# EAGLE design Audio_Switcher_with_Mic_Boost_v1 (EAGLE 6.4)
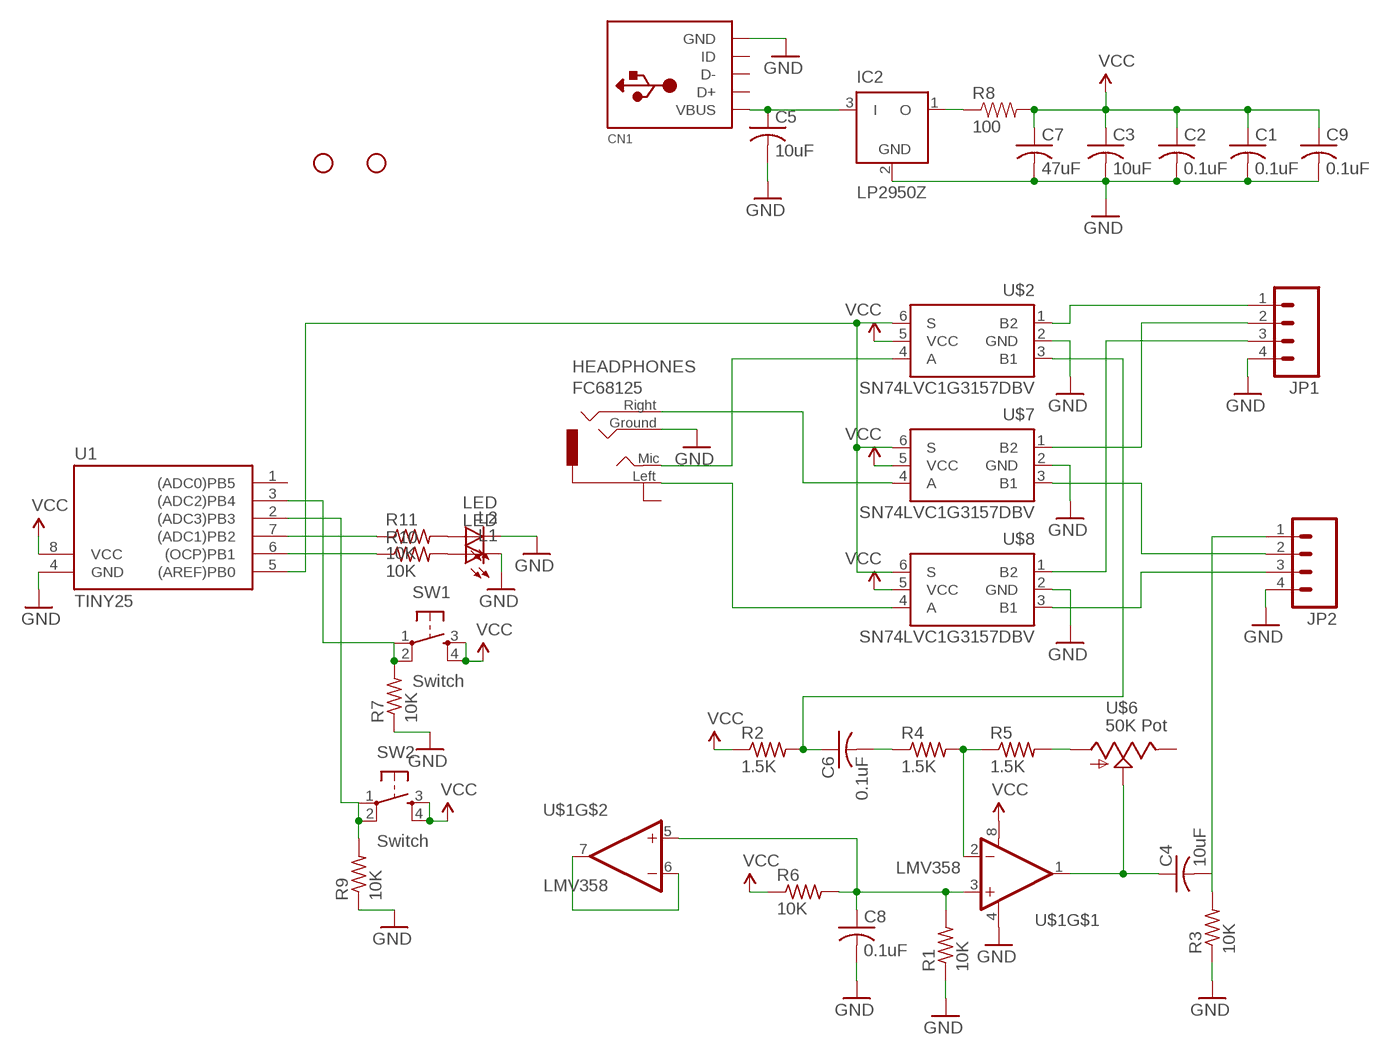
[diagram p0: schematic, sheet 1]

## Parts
C1  0.1uF  C-USC0805K  [C0805K]
C2  0.1uF  C-USC0805K  [C0805K]
C3  10uF  C-US025-024X044  [C025-024X044]
C4  10uF  C-US025-024X044  [C025-024X044]
C5  10uF  C-US025-024X044  [C025-024X044]
C6  0.1uF  C-USC0805K  [C0805K]
C7  47uF  C-US025-024X044  [C025-024X044]
C8  0.1uF  C-USC0805K  [C0805K]
C9  0.1uF  C-USC0805K  [C0805K]
CN1  USBMINIB  [USB-MINIB]
HEADPHONES  FC68125  [FC68125]
IC2  LP2950Z  [TO92]
JP1  M04PTH  [1X04]
JP2  M04PTH  [1X04]
JP3  STAND-OFF2MM  [STAND-OFF-M2]
JP5  STAND-OFF2MM  [STAND-OFF-M2]
L1  LED  LED3MM  [LED3MM]
L2  LED  LED3MM  [LED3MM]
R1  10K  R-US_R0805_2  [R0805_2]
R2  1.5K  R-US_R0805_2  [R0805_2]
R3  10K  R-US_R0805_2  [R0805_2]
R4  1.5K  R-US_R0805_2  [R0805_2]
R5  1.5K  R-US_R0805_2  [R0805_2]
R6  10K  R-US_R0805_2  [R0805_2]
R7  10K  R-US_R0805_2  [R0805_2]
R8  100  RESISTOR5MM  [RESISTOR5MM]
R9  10K  R-US_R0805_2  [R0805_2]
R10  10K  R-US_R0805_2  [R0805_2]
R11  10K  R-US_R0805_2  [R0805_2]
SW1  Switch  TAC_SWITCHPTH  [TACTILE-PTH]
SW2  Switch  TAC_SWITCHPTH  [TACTILE-PTH]
U1  TINY25  [SO08]
U$1  LMV358  LM358SO-08  [SO-08]
U$2  SN74LVC1G3157DBV  [SOT23-DBV-2]
U$6  50K Pot  POT  [ENC_9.6MM]
U$7  SN74LVC1G3157DBV  [SOT23-DBV-2]
U$8  SN74LVC1G3157DBV  [SOT23-DBV-2]

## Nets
GND: C1.2 C2.2 C3.2 C5.2 C7.2 C8.2 C9.2 CN1.GND HEADPHONES.4 IC2.2(GND) JP1.4 JP2.4 L1.K(C) L2.K(C) R1.1 R3.1 R7.1 R9.1 U1.4(GND) U$1.4(V-) U$2.2(GND) U$7.2(GND) U$8.2(GND)
INPUT_LEFT: HEADPHONES.1 U$8.4(A)
INPUT_MIC: HEADPHONES.3 U$2.4(A)
INPUT_RIGHT: HEADPHONES.2 U$7.4(A)
N$1: C4.1 U$1.1(OUT) U$6.C(S)
N$2: C6.1 R2.2 U$2.3(B1)
N$3: JP1.2 U$7.1(B2)
N$4: JP2.2 U$7.3(B1)
N$5: JP2.3 U$8.3(B1)
N$6: JP1.3 U$8.1(B2)
N$7: R5.2 U$6.A
N$10: JP1.1 U$2.1(B2)
N$11: R10.1 U1.6((OCP)PB1)
N$13: R11.1 U1.7((ADC1)PB2)
N$14: L1.A R10.2
N$15: L2.A R11.2
N$16: C8.1 R1.2 R6.2 U$1.3(+IN) U$1.5(+IN)
N$18: R4.2 R5.1 U$1.2(-IN)
N$19: C6.2 R4.1
N$21: C4.2 JP2.1 R3.2
N$22: C5.1 CN1.VBUS IC2.3(I)
N$23: U$1.6(-IN) U$1.7(OUT)
N$24: IC2.1(O) R8.P$1
SELECT: U1.5((AREF)PB0) U$2.6(S) U$7.6(S) U$8.6(S)
SW2: R9.2 SW2.1 SW2.2 U1.2((ADC3)PB3)
VCC: C1.1 C2.1 C3.1 C7.1 C9.1 R2.1 R6.1 R8.P$2 SW1.3 SW1.4 SW2.3 SW2.4 U1.8(VCC) U$1.8(V+) U$2.5(VCC) U$7.5(VCC) U$8.5(VCC)
VCC1: R7.2 SW1.1 SW1.2 U1.3((ADC2)PB4)
Unconnected: CN1.D+ CN1.D- CN1.ID HEADPHONES.5 U1.1((ADC0)PB5) U$6.B(E)

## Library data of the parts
C1-C9 = adafruit:C-US: CAPACITOR, American symbol
CN1 = adafruit:USB: USB Connectors USBMINIB - Surface Mount Female Mini-B USB Connector 4UConnector: 06564 By microbuilder.eu Thru-hole RA Female Mini-B USB Connector 4UConnector: 18732 By ladyada.net
HEADPHONES = SparkFun:FC68125
IC2 = linear:LP2950: 100 mA, Low Power Low Dropout Voltage Regulator Source: http://www.onsemi.com/pub/Collateral/LP2950-D.PDF
JP1 JP2 = SparkFun:M04: Header 4 Standard 4-pin 0.1" header. Use with straight break away headers (SKU : PRT-00116), right angle break away headers (PRT-00553), swiss pins (PRT-00743), machine pins (PRT-00117), and female headers (PRT-00115). Molex polarized connector foot print use with SKU : PRT-08231 with associated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
JP3 JP5 = SparkFun:STAND-OFF: Stand Off
L1 L2 = SparkFun:LED: LEDs
R1-R7 R9-R11 = adafruit:R-US_: RESISTOR, American symbol
R8 = SparkFun:RESISTOR: Resistor
SW1 SW2 = SparkFun:TAC_SWITCH: Momentary Switch Button commonly used for reset or general input. Spark Fun Electronics SKU : COM-00097
U1 = avr-5:TINY25
U$1 = SparkFun:LM358
U$2 U$7 U$8 = texas:SN74LVC1G3157
U$6 = switch-alps_old:POT

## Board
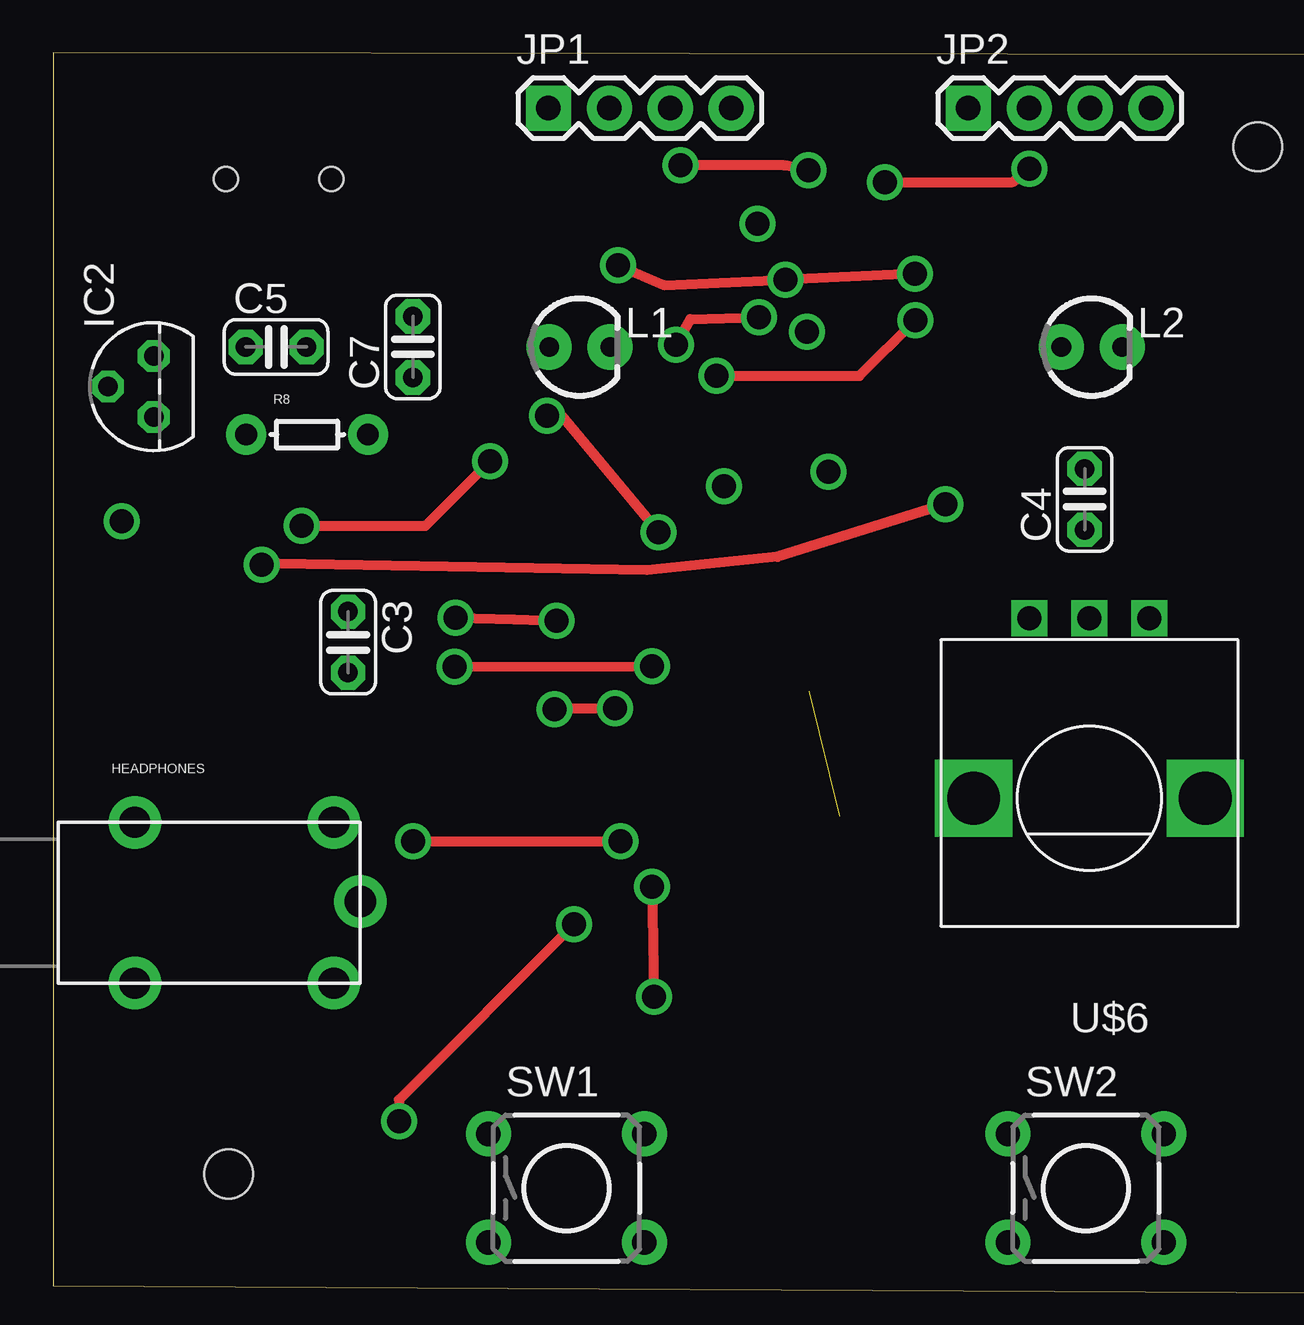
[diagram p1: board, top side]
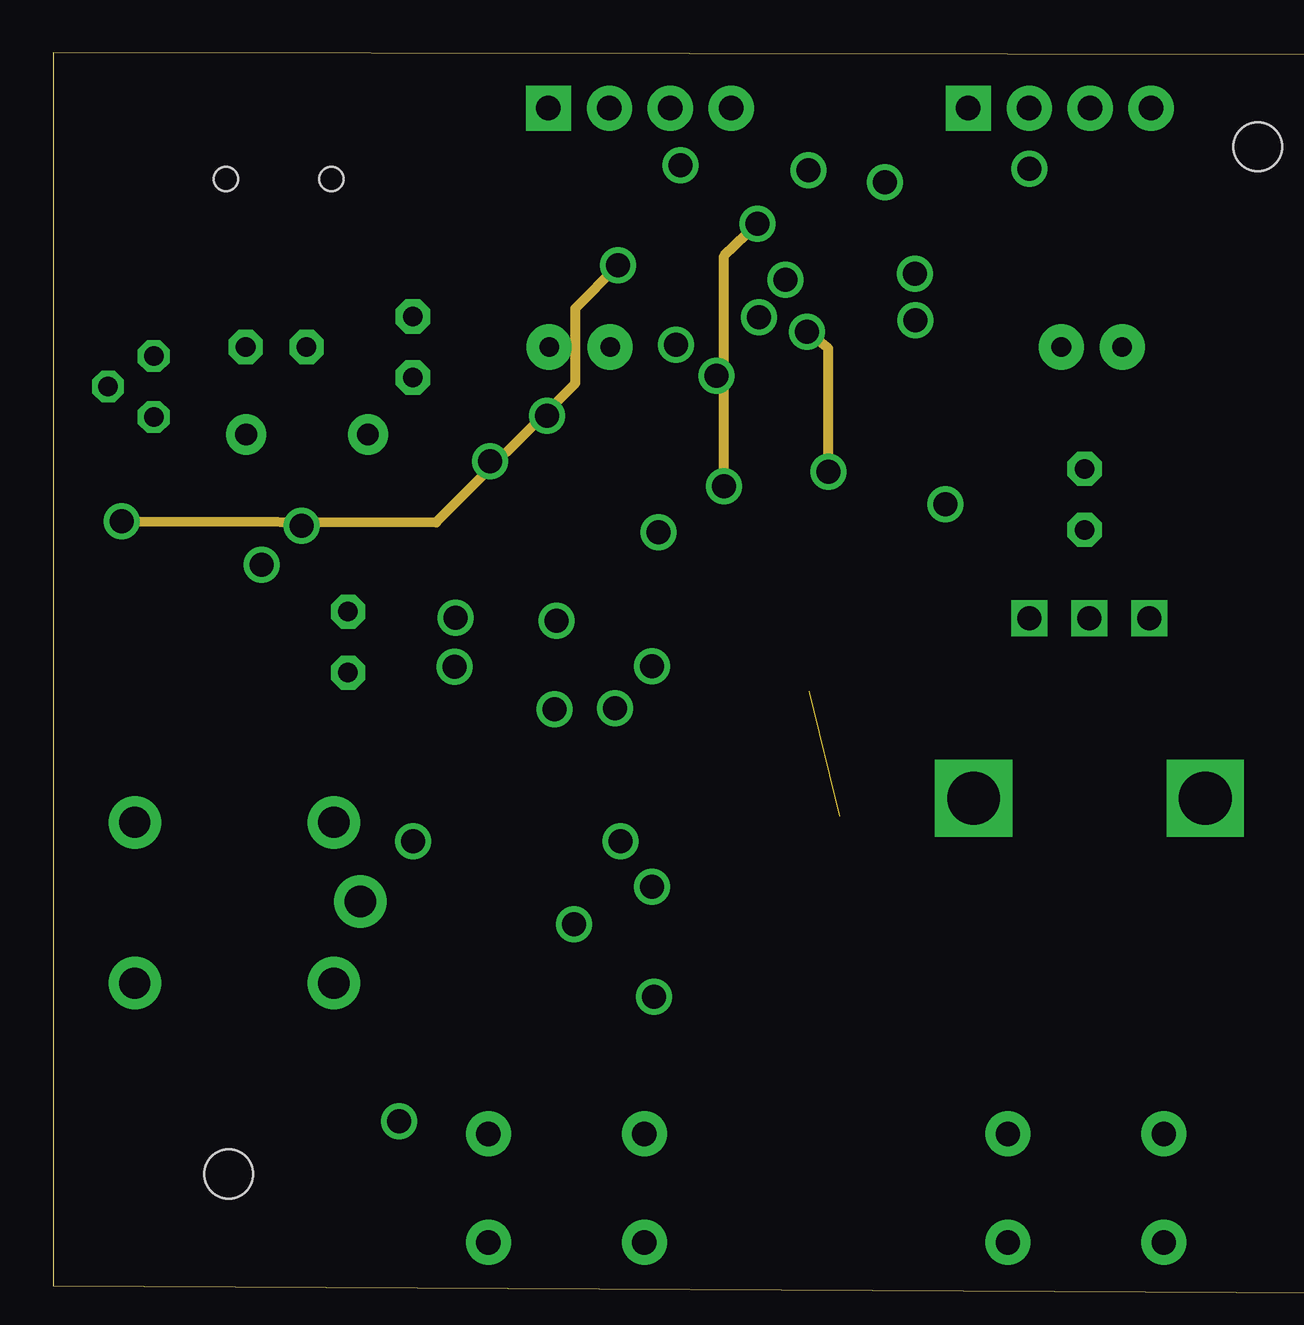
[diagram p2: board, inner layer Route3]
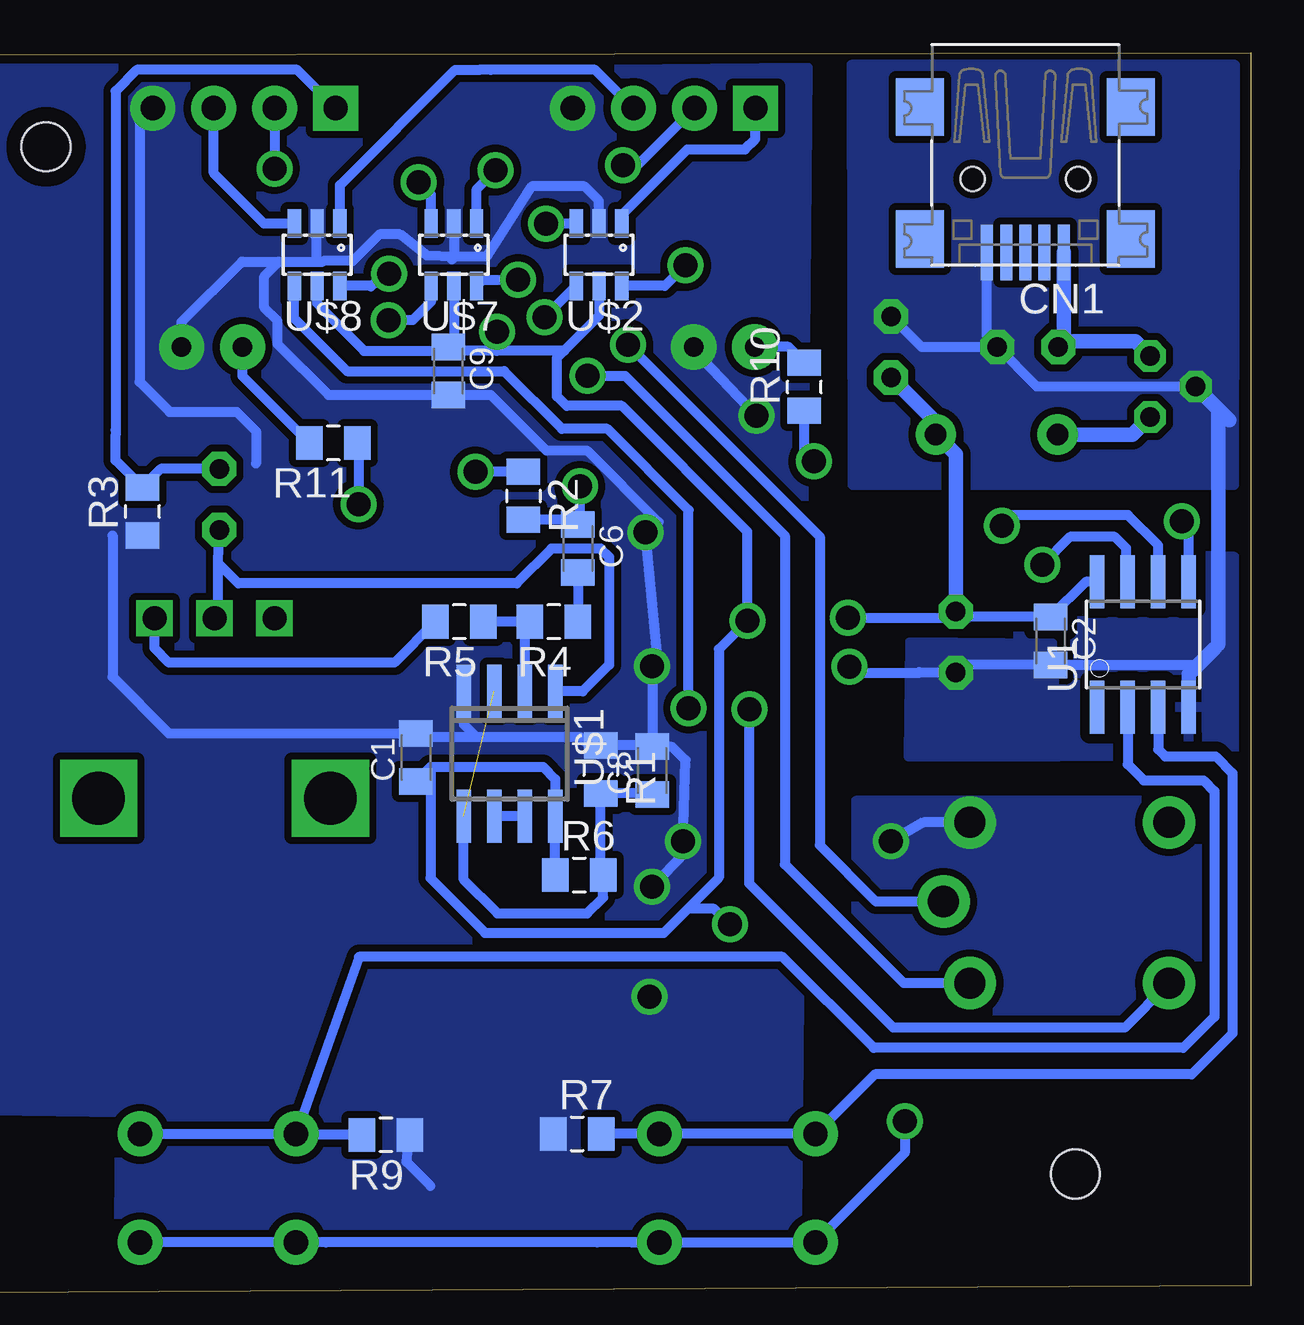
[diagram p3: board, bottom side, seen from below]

No outline drawn. Coordinates in mm, seen from the top.
Copper layers (1*16): Top 0.035mm / dielectric 1.5mm / Bottom 0.035mm
Design rules "ITead_rule": minimum track width 6mil, minimum drill 12mil, track to track 6mil, track to pad 6mil, pad to pad 6mil, via to via 6mil, smd to smd 0mil, copper to edge 10mil, drill to drill 10mil, minimum pad ring 10mil, minimum via ring 6mil, stop-mask expansion 2mil, vias tented up to drill 100mil, thermal gap 10mil
Milling: 4 lines

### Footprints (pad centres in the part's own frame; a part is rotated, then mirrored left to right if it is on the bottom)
C0805K = smd 1.1 x 1.4: 1 -1,0; 2 1,0
C025-024X044 = drill 0.813 pad 1.422 octagon: 1 -1.27,0; 2 1.27,0
USB-MINIB = smd 0.5 x 2.308: D+ 0,4.064; D- -0.8,4.064; GND 1.6,4.064; ID 0.8,4.064; VBUS -1.6,4.064 | smd 2 x 2.4: GND1 -4.4,-2; GND2 -4.4,3.5; GND3 4.4,3.5; GND4 4.4,-2 | hole 1: -2.2,1; 2.2,1
FC68125 = drill 1.3 pad 2.184: 1 -2.84,-3.66; 2 5.46,-3.66; 3 6.56,-0.26; 4 5.46,3.04; 5 -2.84,3.04
TO92 = drill 0.813 octagon: 1 -1.27,0; 2 0,1.905; 3 1.27,0
1X04 = drill 1.016 pad 1.88 square: 1 0,0 | drill 1.016 pad 1.88: 2 2.54,0; 3 5.08,0; 4 7.62,0
STAND-OFF-M2 = hole 2.032: 0,0
LED3MM = drill 0.813 pad 1.88: A -1.27,0; K 1.27,0
R0805_2 = smd 1.1 x 1.4: 1 -1,0; 2 1,0
RESISTOR5MM = drill 0.9 pad 1.676: P$1 -2.5,0; P$2 2.58,0
TACTILE-PTH = drill 1.016 pad 1.88: 1 -3.251,2.261; 2 3.251,2.261; 3 -3.251,-2.261; 4 3.251,-2.261
SO08 = smd 0.61 x 2.21: 1 -1.905,-2.616; 2 -0.635,-2.616; 3 0.635,-2.616; 4 1.905,-2.616; 5 1.905,2.616; 6 0.635,2.616; 7 -0.635,2.616; 8 -1.905,2.616
SO-08 = smd 0.6 x 2.2: 1 -1.905,-2.6; 2 -0.635,-2.6; 3 0.635,-2.6; 4 1.905,-2.6; 5 1.905,2.6; 6 0.635,2.6; 7 -0.635,2.6; 8 -1.905,2.6
SOT23-DBV-2 = smd 0.55 x 1.2: 1 -0.95,-1.3; 2 0,-1.3; 3 0.95,-1.3; 4 0.95,1.3; 5 0,1.3; 6 -0.95,1.3
ENC_9.6MM = drill 1 square: A -2.5,-7.5; B 2.5,-7.5; C 0,-7.5 | drill 2.2 square: GND1 -4.83,0; GND2 4.83,0

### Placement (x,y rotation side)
C1  34.78,-29.24 90 bottom
C2  8.33,-24.39 270 bottom
C3  12.28,-24.44 270 top
C4  42.98,-18.49 90 top
C5  9.28,-12.14 0 top
C6  28.03,-20.54 270 bottom
C7  14.98,-12.14 90 top
C8  24.93,-29.79 90 bottom
C9  33.43,-13.14 270 bottom
CN1  9.38,-4.14 180 bottom
HEADPHONES  6.23,-34.99 0 top
IC2  4.18,-13.79 90 top
JP1  20.63,-2.19 0 top
JP2  38.13,-2.19 0 top
JP3  7.3,-46.6 0 top
JP5  50.2,-3.8 0 top
L1  21.93,-12.14 0 top
L2  43.28,-12.14 0 top
R1  27.08,-29.74 270 bottom
R2  30.3,-18.34 270 bottom
R3  46.18,-18.99 90 bottom
R4  29.03,-23.59 180 bottom
R5  32.98,-23.59 180 bottom
R6  27.98,-34.14 0 bottom
R7  28.06,-44.93 0 bottom
R8  10.53,-15.79 0 top
R9  36.04,-44.97 180 bottom
R10  18.59,-13.8 90 bottom
R11  38.23,-16.14 180 bottom
SW1  21.38,-47.19 0 top
SW2  43.03,-47.19 0 top
U1  4.48,-24.54 0 bottom
U$1  30.88,-29.09 180 bottom
U$2  27.15,-8.3 180 bottom
U$6  43.18,-30.94 180 top
U$7  33.2,-8.3 180 bottom
U$8  38.9,-8.3 180 bottom

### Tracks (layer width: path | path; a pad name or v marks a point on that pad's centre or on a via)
GND  (via drill 1)
  Top 0.406: v16.71,-25.47 v24.95,-25.44 | v14.99,-32.73 v23.64,-32.73 | v20.58,-15 21.17,-15.01 v25.21,-19.86 | v24.95,-34.63 v25.04,-39.21
  Bottom 0.406: C5.2 10.98,-11.71 CN1.GND | IC2.2 8.9,-13.79 C5.2 | C7.2 13.71,-12.14 C5.2 | 47.43,-19.99 47.43,-25.89 45.08,-28.24 C1.2 | R1.1 27.58,-28.75 | U$1.4 32.78,-27.86 32.25,-28.4 | 35.18,-28.24 C1.2 | 2.58,-25.79 U1.4 | 13.78,-25.71 C3.2 11.96,-25.39 C2.2 2.18,-25.39 1.5,-24.71 | C8.2 24.98,-28.75 27.58,-28.75 | 34.18,-47.09 35.18,-46.09 R9.1 | HEADPHONES.4 13.62,-31.95 v14.99,-32.73 | 13.8,-25.69 13.78,-25.71 | L1.K 23.2,-12.25 v20.58,-15 | 33.2,-8.38 31.84,-8.38 29.96,-5.45 27.75,-5.45 27.15,-6.05 U$2.2 | 33.28,-8.5 33.2,-8.38 | 40.5,-8.58 42.03,-8.58 44.55,-11.1 L2.K | 40.5,-8.58 38.95,-8.58 | 38.95,-8.58 38.65,-8.58 38.62,-8.55 37.4,-8.55 36.3,-7.45 35.45,-7.45 34.32,-8.33 33.2,-8.38 | C8.2 24.93,-25.77 v24.95,-25.44 24.66,-25.5 v25.21,-19.86 24.66,-19.43 27.65,-16.45 29.35,-16.45 31.66,-14.14 C9.2 38.43,-14.14 40.55,-12.02 40.55,-11.05 41.1,-10.5 41.1,-9.2 40.5,-8.6 40.5,-8.58 | 27.58,-28.75 27.93,-28.4 32.25,-28.4 | 32.25,-28.4 34.62,-28.4 C1.2 | C8.2 24.1,-28.8 23.54,-29.36 v23.64,-32.73 23.54,-33.17 v24.95,-34.63 | JP2.4 46.3,-2.74 46.3,-13.6 45.05,-14.85 42.25,-14.85 41.45,-15.65 41.45,-17 | 33.28,-7 U$7.2 33.2,-8.38 | U$8.2 38.95,-7.05 38.95,-8.58 | v16.71,-25.47 16.47,-25.71 13.78,-25.71
  Bottom 0.61: IC2.2 1.33,-14.74 | 1.33,-14.74 0.88,-15.19 | 1.33,-14.74 1.33,-24.54 1.5,-24.71 2.58,-25.79 U1.4
  pour Bottom (isolate 0.305, no thermals): 0.63,-0.39 16.63,-0.39 16.58,-17.89 0.68,-17.89
  pour Bottom (isolate 0.406): 0.66,-20.89 9.69,-20.5 9.7,-29.17 0.68,-29.19
  pour Bottom (no thermals): 8.25,-24.5 14.2,-24.45 14.25,-29.2 8,-29.2
  pour Bottom (isolate 0.305, no thermals): 18.45,-0.5 46.7,-0.8 47.2,-50.7 18.9,-50.65
  pour Bottom (isolate 0.305, no thermals): 0.9,-31.05 16.45,-31.05 16.45,-40.8 1,-41.05
  pour Bottom (isolate 0.305, no thermals): 38.45,-0.5 52.35,-0.55 52.6,-43.95 38.55,-44.15
INPUT_LEFT  (via drill 1)
  Top 0.406: v20.88,-27.24 20.93,-27.19 v23.41,-27.19
  Bottom 0.406: HEADPHONES.1 5.24,-40.5 14.88,-40.5 20.88,-34.5 v20.88,-27.24 | v23.41,-27.19 23.41,-18.94 26.8,-15.55 28.7,-15.55 31.1,-13.15 37.65,-13.15 39.85,-10.95 U$8.4
INPUT_MIC  (via drill 1)
  Top 0.406: v25.95,-12.04 26.55,-10.98 v29.41,-10.91
  Bottom 0.406: U$2.4 v29.41,-10.91 | v25.95,-12.04 17.95,-20.04 17.95,-32.9 15.6,-35.25 HEADPHONES.3
INPUT_RIGHT  (via drill 1)
  Top 0.406: v27.63,-13.34 33.6,-13.34 v35.92,-11.02
  Bottom 0.406: v35.92,-11.02 34.91,-11.02 34.15,-10.26 U$7.4 | v27.63,-13.34 26.06,-13.34 19.4,-20 19.4,-33.7 14.45,-38.65 HEADPHONES.2
N$1
  Bottom 0.406: U$1.1 27.83,-26.49 26.73,-25.39 26.73,-20.89 27.08,-20.54 29.13,-20.54 30.58,-21.99 42.19,-21.99 43.03,-21.15 | U$6.C 43.03,-23.29 43.03,-21.15 | 43.03,-21.15 C4.1
N$2  (via drill 1)
  Route3 0.406: v27.95,-17.95 27.95,-8.35 v29.35,-7
  Bottom 0.406: C6.1 28.23,-19.34 | 28.23,-19.34 R2.2 | U$2.3 v29.35,-7 | 28.23,-19.34 27.95,-19.06 v27.95,-17.95
N$3  (via drill 1)
  Top 0.406: v31.46,-4.77 30.46,-4.57 v26.14,-4.57
  Bottom 0.406: v26.14,-4.57 25.55,-4.57 JP1.2 | U$7.1 32.25,-5.56 v31.46,-4.77
N$4  (via drill 1)
  Top 0.406: v34.66,-5.27 39.97,-5.27 v40.68,-4.71
  Bottom 0.406: JP2.2 v40.68,-4.71 | U$7.3 34.15,-5.78 v34.66,-5.27
N$5
  Bottom 0.406: JP2.3 43.21,-4.9 41.11,-7 U$8.3
N$6
  Bottom 0.406: JP1.3 27.31,-0.59 31.65,-0.59 32.14,-0.59 33.14,-0.59 37.95,-5.4 U$8.1 37.98,-6.9
N$7
  Bottom 0.406: R5.2 35.68,-25.29 45.08,-25.29 45.68,-24.69 U$6.A
N$10
  Bottom 0.406: JP1.1 20.63,-3.48 21.06,-3.91 23.47,-3.91 26.2,-6.64 U$2.1 26.2,-7.04
N$11  (via drill 1)
  Top 0.406: v10.35,-19.6 15.5,-19.6 v18.2,-16.9
  Bottom 0.406: U1.6 3.85,-20.41 5.1,-19.15 9.9,-19.15 v10.35,-19.6 | v18.2,-16.9 18.59,-16.51 R10.1
N$13  (via drill 1)
  Top 0.406: v37.18,-18.69 30.18,-20.89 24.73,-21.44 9.35,-21.17 v8.68,-21.21
  Bottom 0.406: U1.7 5.18,-21.86 5.18,-20.52 5.65,-20.05 7.52,-20.05 v8.68,-21.21 | R11.1 37.18,-16.19 v37.18,-18.69
N$14
  Bottom 0.406: R10.2 19.25,-12.14 L1.A
N$15
  Bottom 0.406: R11.2 42.01,-13.36 L2.A
N$16  (1 unrouted)
  Bottom 0.406: U$1.5 32.78,-34.34 31.38,-35.74 27.64,-35.74 26.98,-35.08 R6.2 26.93,-34.09 27.08,-33.94 R1.2 24.98,-30.74 C8.1
N$18
  Bottom 0.406: R5.1 R4.2 30.25,-23.8 U$1.2
N$19
  Bottom 0.406: C6.2 R4.1
N$21
  Bottom 0.406: JP2.1 39.73,-0.59 46.41,-0.59 47.3,-1.48 47.3,-15.6 47.3,-15.82 47.3,-16.87 R3.2 45.41,-17.22 C4.2
N$22
  Bottom 0.61: CN1.VBUS 7.78,-11.91 | 7.78,-11.91 C5.1 | 7.78,-11.91 4.79,-11.91 IC2.3
N$23
  Bottom 0.406: U$1.7 U$1.6
N$24
  Bottom 0.61: IC2.1 4.91,-15.79 R8.P$1
SELECT  (via drill 1)
  Top 0.406: v35.9,-9.08 v30.52,-9.34 25.46,-9.56 v23.54,-8.74
  Route3 0.406: v2.85,-19.4 15.95,-19.45 21.75,-13.65 21.75,-10.53 v23.54,-8.74
  Bottom 0.406: v35.9,-9.08 36.66,-9.62 36.68,-9.6 U$8.6 37.95,-9.62 | U1.5 2.58,-19.68 v2.85,-19.4 | v23.54,-8.74 24.4,-9.6 U$2.6 | U$7.6 31.99,-9.34 v30.52,-9.34
SW2
  Bottom 0.406: SW2.2 SW2.1 | SW2.1 37.15,-37.55 19.5,-37.55 15.7,-41.35 2.8,-41.35 1.5,-40.05 1.5,-30.65 1.95,-30.2 4.45,-30.2 5.12,-29.54 U1.2 | R9.2 39.78,-44.97 SW2.1
VCC  (via drill 1)
  Top 0.406: v16.77,-23.43 19.21,-23.49 v20.96,-23.54 | v21.7,-36.2 14.4,-43.5 v14.4,-44.4
  Route3 0.406: v32.3,-17.35 32.3,-12.2 v31.4,-11.5
  Bottom 0.406: C1.1 34.18,-29.64 | 34.18,-29.64 29.48,-29.64 28.98,-30.14 U$1.8 | U$1.8 28.93,-31.73 | R6.1 U$1.8 | U1.8 6.86,-21.92 C2.1 11.75,-23.39 | 11.75,-23.39 12.33,-23.39 12.28,-23.34 C3.1 | 33.59,-12.3 36.95,-12.3 38.65,-10.6 38.63,-10.58 38.9,-10.31 U$8.5 38.9,-9.2 | 28.6,-12.3 27.15,-10.85 U$2.5 | 28.6,-12.3 31.4,-12.3 | 31.4,-12.3 33.59,-12.3 | C9.1 33.59,-12.3 | 33.28,-11.99 C9.1 | 28.6,-12.3 28.9,-12.6 28.9,-14.2 28.5,-14.6 26.2,-14.6 20.96,-19.84 v20.96,-23.54 22.15,-24.73 22.15,-34.25 23.45,-35.55 | 34.18,-29.64 34.18,-34.27 31.9,-36.55 24.45,-36.55 23.45,-35.55 | v16.77,-23.43 11.79,-23.43 11.75,-23.39 | R2.1 v32.29,-17.34 v32.3,-17.35 | v31.4,-11.5 31.4,-12.3 | 33.28,-9.6 U$7.5 33.2,-11.91 C9.1 | 25.79,-49.45 SW1.4 | SW1.4 SW1.3 14.4,-45.72 v14.4,-44.4 | SW1.4 27.22,-49.45 | SW2.3 SW2.4 | 38.54,-49.45 SW2.3 | SW1.4 SW2.3 | SW1.4 22.2,-49.45 | v21.7,-36.2 22.35,-35.55 23.45,-35.55
  Bottom 0.61: C7.1 13.11,-15.28 R8.P$2 12.28,-16.62 C3.1
VCC1
  Bottom 0.406: U1.3 3.85,-28.91 3.55,-29.2 1.45,-29.2 0.75,-29.9 0.75,-40.75 2.45,-42.45 15.65,-42.45 SW1.1 SW1.2 R7.2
